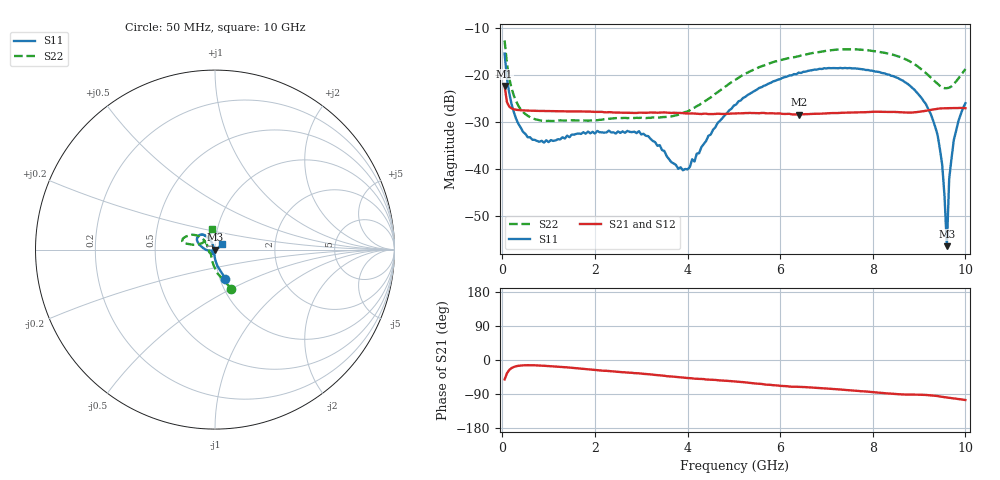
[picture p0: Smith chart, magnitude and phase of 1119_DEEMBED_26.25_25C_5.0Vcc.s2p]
!Hittite Microwave Corp.
!Digital Attenuator/PhaseShifter Rev 1.4.0
!Filename: C:\DATA\DATA\1119_DEEMBED_26.25_25C_5.0Vcc.s2p
!VNA ID: Agilent Technologies,N5224A,MY51441122,A.10.45.03
!Device type:
!2 Port Calibration.
!Temp(C): 25
!Lot Number:
!Serial Number:
!Operator:
!Misc:
!Attenuator:  26.250
# GHZ S DB R 50.0
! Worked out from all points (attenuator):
!   200 points, 50 MHz to 10 GHz, reference 50 ohm
!   highest |S21| = -22.29 dB at 50 MHz (marker M1); lowest = -28.4 dB at 6.4 GHz (marker M2)
!   lowest |S11| = -56.5 dB at 9.6 GHz (marker M3), VSWR 1.00, Z = 50.1 - j0.0716 ohm
!   |S11| at or under -10 dB: start of sweep to end of sweep
!   |S22| runs from -29.8 to -12.6 dB; largest |S21 - S12| = 0.00015
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0.05  -15.35 -70.6  -22.29 -51.3  -22.30 -51.3  -12.56 -67.3
0.1  -20.62 -81.4  -25.74 -35.2  -25.74 -35.2  -17.51 -83.9
0.2  -26.16 -90.3  -27.08 -21.3  -27.08 -21.1  -22.79 -100.5
0.55  -33.25 -104.6  -27.55 -13.7  -27.55 -13.7  -28.67 -126.3
1.75  -32.17 -120.7  -27.75 -23.3  -27.74 -23.4  -29.66 -140.7
2.95  -31.95 -116.9  -27.99 -35.2  -28.00 -35.3  -29.12 -159.9
3.4  -34.94 -129.9  -27.98 -40.3  -27.99 -40.4  -29.03 -173.5
3.8  -40.00 -165.4  -28.06 -45.5  -28.06 -45.5  -28.45 170.6
4  -40.12 157.3  -28.17 -47.5  -28.18 -47.6  -27.75 162.2
5.05  -26.26 115.1  -28.16 -56.9  -28.17 -56.9  -20.83 138.8
6.4  -19.43 128.6  -28.39 -70.9  -28.41 -71.0  -15.93 149.9
6.7  -18.89 133.4  -28.25 -72.8  -28.26 -72.8  -15.25 153.9
8.35  -19.86 158.1  -27.84 -88.3  -27.84 -88.4  -15.40 168.1
8.9  -23.09 170.6  -27.93 -91.2  -27.94 -91.2  -17.62 167.6
9.3  -29.59 -170.2  -27.33 -93.9  -27.34 -93.9  -20.89 160.1
9.400001  -32.78 -165.1  -27.17 -95.2  -27.18 -95.2  -21.83 153.6
9.5  -39.19 -160.7  -27.07 -97.2  -27.08 -97.2  -22.60 143.9
9.55  -45.98 -141.0  -27.05 -98.1  -27.05 -98.1  -22.75 138.2
9.6  -56.53 -28.6  -27.04 -98.9  -27.05 -98.9  -22.77 132.3
9.65  -42.16 15.2  -27.03 -99.7  -27.03 -99.7  -22.65 126.1
9.75  -33.82 28.2  -27.01 -101.3  -27.02 -101.3  -21.91 114.2
10  -25.97 41.9  -27.03 -105.6  -27.04 -105.6  -18.67 98.5
